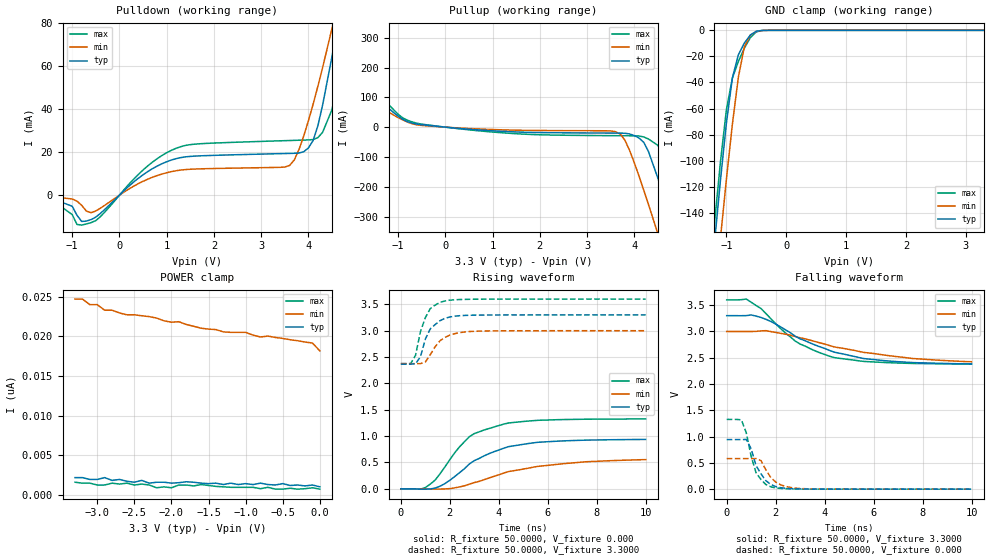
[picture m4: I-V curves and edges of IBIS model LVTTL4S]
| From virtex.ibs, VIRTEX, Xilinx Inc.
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|   Model LVTTL4S
[Model]   LVTTL4S
Model_type   I/O
Polarity   Non-Inverting
Enable   Active-Low
Vinl =   0.800V
Vinh =   2.000V
Vmeas =   1.4000V
Cref =  35.0000pF
Rref =   1.0000M
Vref =  0.000V
C_comp   6.5000pF   5.0000pF   8.0000pF
[Temperature Range]   27.0000   100.0000   0.000
[Voltage Range]   3.3000V   3.0000V   3.6000V
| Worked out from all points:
|   slope of the pulldown table from 0 to 0.495 V, typ, clamps not added: 52.7 ohm
|   slope of the pullup table from 0 to 0.495 V, typ, clamps not added: 72 ohm
|   GND clamp passes 1 mA (typ) near -0.51 V on its own axis
|   rising waveform, R_fixture 50.0000, V_fixture 0.000: 20-80 % time 2.01ns typ, 3.02ns min, 1.51ns max; typ from 0 V to 0.937 V
|   rising waveform, R_fixture 50.0000, V_fixture 3.3000: 20-80 % time 564ps typ, 671ps min, 487ps max; typ from 2.37 V to 3.3 V
|   falling waveform, R_fixture 50.0000, V_fixture 3.3000: 20-80 % time 2.73ns typ, 3.68ns min, 2.08ns max; typ from 3.3 V to 2.38 V
|   falling waveform, R_fixture 50.0000, V_fixture 0.000: 20-80 % time 550ps typ, 587ps min, 467ps max; typ from 0.943 V to 0 V
[Pulldown]
| voltage   I(typ)   I(min)   I(max)
-3.3V     0A         0A         -1mA
-1.5V     -1mA       -500uA     -1.2mA
-800mV    -12.23mA   -4.72mA    -13.9mA
-600mV    -11.34mA   -8.171mA   -12.78mA
1.2V      16.95mA    11.33mA    21.76mA
3.6V      19.37mA    13.78mA    25.36mA
3.8V      19.56mA    21.23mA    25.5mA
4.1V      25.44mA    42.35mA    25.81mA
4.5V      64.6mA     77.61mA    39.82mA
4.7V      89.71mA    97.03mA    64.96mA
4.9V      116.1mA    117.3mA    95.67mA
6.6V      348mA      295mA      376.7mA
[Pullup]
| voltage   I(typ)   I(min)   I(max)
-3.3V     354.4mA    271.9mA    429.9mA
-2.7V     272.8mA    207.8mA    331mA
-800mV    18.43mA    17.03mA    23.04mA
3.6V      -19.96mA   -15.22mA   -28.65mA
3.8V      -20.52mA   -43.41mA   -28.84mA
4.2V      -51mA      -211.2mA   -32.92mA
4.5V      -171.4mA   -357.8mA   -61.08mA
4.7V      -272mA     -457.9mA   -116mA
4.9V      -376.2mA   -559mA     -210.3mA
5.1V      -482.2mA   -660.7mA   -313.6mA
5.3V      -589.2mA   -762.8mA   -420.3mA
6.6V      -1.293A    -1.432A    -1.133A
[GND_clamp]
| voltage   I(typ)   I(min)   I(max)
-3.3V     -1.286A    -1.273A    -1.289A
-1.2V     -163.3mA   -206.7mA   -148.3mA
-1.1V     -115.2mA   -159.6mA   -101mA
-1V       -71.04mA   -114.2mA   -60.78mA
-900mV    -36.42mA   -71.86mA   -36.53mA
-800mV    -18.72mA   -35.86mA   -23.84mA
-700mV    -9.715mA   -12.62mA   -13.63mA
-600mV    -3.608mA   -3.649mA   -5.602mA
-500mV    -692.7uA   -854.2uA   -1.156mA
-400mV    -68.48uA   -138.7uA   -98.54uA
-300mV    -4.365uA   -16.73uA   -4.627uA
3.3V      1.106nA    19.5nA     40.4nA
[POWER_clamp]
| voltage   I(typ)   I(min)   I(max)
-3.3V     2.212nA    24.68nA    1.63nA
-3.2V     2.212nA    24.68nA    1.513nA
-3.1V     1.979nA    23.98nA    1.513nA
-3V       1.979nA    23.98nA    1.281nA
-2.9V     2.212nA    23.28nA    1.281nA
-2.6V     1.746nA    22.7nA     1.513nA
-2.3V     1.513nA    22.47nA    1.281nA
-2.2V     1.63nA     22.29nA    931.3pA
-1.6V     1.513nA    21.01nA    1.339nA
-600mV    1.281nA    19.85nA    756.7pA
-100mV    1.281nA    19.15nA    931.3pA
0V        1.048nA    18.16nA    756.7pA
[Ramp]
| variable   typ   min   max
dV/dt_r   0.5622/2.0206n   0.3323/2.9769n   0.7950/1.5333n
dV/dt_f   0.5508/2.7270n   0.3456/3.6283n   0.7320/2.0742n
R_load = 50.0000
[Rising Waveform]
R_fixture = 50.0000
V_fixture = 0.000
| time   V(typ)   V(min)   V(max)
0s        0V         0V         0V
1ns       -5.859mV   -1.95mV    24.41mV
1.4ns     14.65mV    -5.822mV   166.1mV
1.8ns     99.94mV    -1.623mV   416.7mV
2.4ns     307.7mV    36.82mV    798.3mV
2.8ns     472.4mV    89.52mV    989.3mV
4.2ns     770.7mV    298.6mV    1.228V
5.6ns     882.9mV    426.6mV    1.3V
7.6ns     924.3mV    514.6mV    1.321V
10ns      937mV      553.8mV    1.325V
[Rising Waveform]
R_fixture = 50.0000
V_fixture = 3.3000
V_fixture_min = 3.0000
V_fixture_max = 3.6000
| time   V(typ)   V(min)   V(max)
0s        2.365V     2.374V     2.375V
400ps     2.365V     2.374V     2.375V
600ps     2.373V     2.374V     2.532V
800ps     2.503V     2.374V     2.98V
1ns       2.839V     2.404V     3.247V
1.2ns     3.032V     2.544V     3.417V
1.6ns     3.189V     2.808V     3.536V
1.8ns     3.233V     2.873V     3.563V
3ns       3.294V     2.988V     3.596V
10ns      3.299V     2.999V     3.599V
[Falling Waveform]
R_fixture = 50.0000
V_fixture = 3.3000
V_fixture_min = 3.0000
V_fixture_max = 3.6000
| time   V(typ)   V(min)   V(max)
0s        3.3V       3V         3.6V
800ps     3.301V     3V         3.616V
1ns       3.314V     2.999V     3.556V
1.6ns     3.231V     3.015V     3.342V
2.8ns     2.909V     2.903V     2.817V
3.6ns     2.744V     2.809V     2.633V
4.4ns     2.605V     2.705V     2.502V
5.6ns     2.485V     2.602V     2.43V
6.6ns     2.438V     2.541V     2.406V
10ns      2.382V     2.424V     2.38V
[Falling Waveform]
R_fixture = 50.0000
V_fixture = 0.000
| time   V(typ)   V(min)   V(max)
0s        943.3mV    581.6mV    1.327V
600ps     943.5mV    581.6mV    1.32V
800ps     944.6mV    581.7mV    1.073V
1ns       768.5mV    581.9mV    624.7mV
1.2ns     447mV      582.5mV    311.4mV
1.4ns     292mV      543.9mV    184.9mV
1.8ns     90.22mV    221.4mV    44.92mV
2.2ns     28.84mV    83.5mV     14.21mV
3ns       4.552mV    12.04mV    3.466mV
10ns      359.8uV    293.3uV    372.9uV
